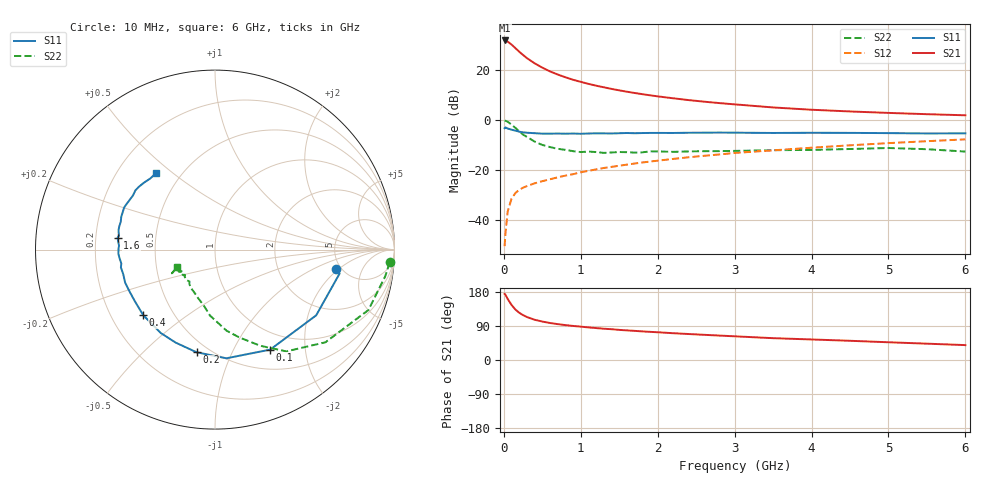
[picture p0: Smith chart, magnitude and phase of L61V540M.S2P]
!  INFINEON TECHNOLOGIES Small Signal Semiconductors
! BFR380L3 , Si-NPN RF-Transistor in TSLP-3-1
!  Vce=1.5 V,  Ic=40 mA
! Common Emitter S-Parameters:  07. March 2005
#  GHz  S  MA  R  50
! f  S11  S21  S12  S22
! GHz  Mag  Ang  Mag  Ang  Mag  Ang  Mag  Ang
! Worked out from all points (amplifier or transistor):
!   36 points, 10 MHz to 6 GHz, reference 50 ohm
!   highest |S21| = 31.7 dB at 10 MHz (marker M1)
!   |S21| within 3 dB of that: start of sweep to 148.2 MHz
!   unconditionally stable (mu >= 1): 1.624 GHz to 4.959 GHz
!   at 250 MHz: K = 0.44, MSG = 26.5 dB, |S12| = -27.1 dB
!   at 1.4 GHz: K = 0.98, MSG = 15.6 dB, |S12| = -18.8 dB
!   at 6 GHz: K = 0.98, MSG = 4.8 dB, |S12| = -7.8 dB
!   S11 on the Smith chart (normalised r, x): 10 MHz: 4.51, -1.84; 100 MHz: 0.75, -1.41; 200 MHz: 0.43, -0.74; 400 MHz: 0.34, -0.35; 1.6 GHz: 0.29, +0.06; 6 GHz: 0.37, +0.44
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0.01  0.6824 -9.2  38.59 174.4  0.003 82.2  0.9755 -4.2
0.02  0.7069 -10.9  38.25 172.5  0.0052 83.3  0.9605 -8.8
0.05  0.6722 -33.0  36.58 161.0  0.0148 76.4  0.9187 -21.5
0.1  0.6365 -61.1  31.93 145.3  0.0267 65.5  0.8033 -40.0
0.15  0.6089 -84.0  27.16 133.2  0.0345 57.7  0.6923 -55.0
0.2  0.5811 -100.2  22.99 124.6  0.0401 54.5  0.5921 -64.8
0.25  0.5627 -112.9  19.78 118.4  0.0441 51.4  0.5078 -74.5
0.3  0.5544 -123.1  17.13 113.4  0.0476 51.0  0.4569 -81.8
0.4  0.5416 -137.6  13.48 106.2  0.054 51.1  0.3689 -94.3
0.5  0.531 -147.6  11.06 101.5  0.0596 52.4  0.3153 -101.8
0.6  0.5305 -154.7  9.293 97.6  0.0651 53.9  0.2862 -109.2
0.7  0.5334 -159.8  8.062 94.7  0.0711 55.8  0.2641 -116.2
0.9  0.5336 -169.3  6.326 89.9  0.0823 58.5  0.2371 -127.2
1.1  0.5341 -174.9  5.237 86.0  0.096 60.4  0.2328 -132.8
1.3  0.5374 179.4  4.473 82.5  0.1094 61.6  0.219 -140.4
1.6  0.5468 173.1  3.652 78.1  0.1278 62.7  0.2263 -146.6
2.2  0.5475 163.6  2.701 70.7  0.1659 63.7  0.2297 -149.0
2.8  0.5577 155.1  2.165 64.5  0.2038 63.7  0.2377 -154.2
3.5  0.5476 146.7  1.771 57.6  0.2463 61.8  0.2481 -152.9
4.5  0.5499 140.5  1.473 50.7  0.3104 60.0  0.2619 -152.1
5.5  0.5357 132.4  1.299 43.1  0.3752 55.9  0.2595 -152.4
6  0.5383 127.4  1.235 39.3  0.4082 53.7  0.2327 -155.9
